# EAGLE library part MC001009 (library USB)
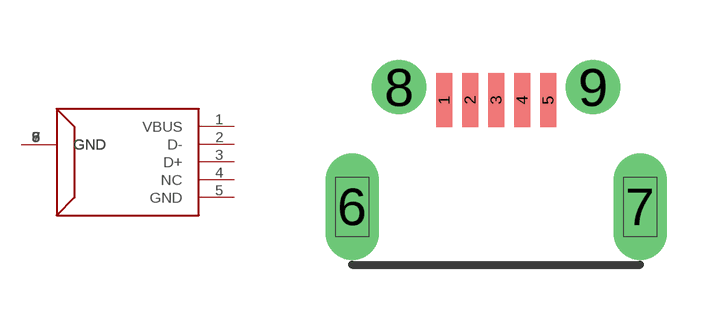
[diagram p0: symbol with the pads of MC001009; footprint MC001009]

Designator prefix U

## MC001009  [MC001009]
1  VBUS
2  D-
3  D+
4  NC
5  GND
6  GND
7  GND
8  GND
9  GND

## Footprint MC001009 (pad centres in mm)
smd 0.4 x 1.35: 1 2.3,2.675; 2 2.95,2.675; 3 3.6,2.675; 4 4.25,2.675; 5 4.9,2.675
drill 0.83 long: 6 0,0; 7 7.2,0
drill 0.85: 8 1.175,3; 9 6.025,3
